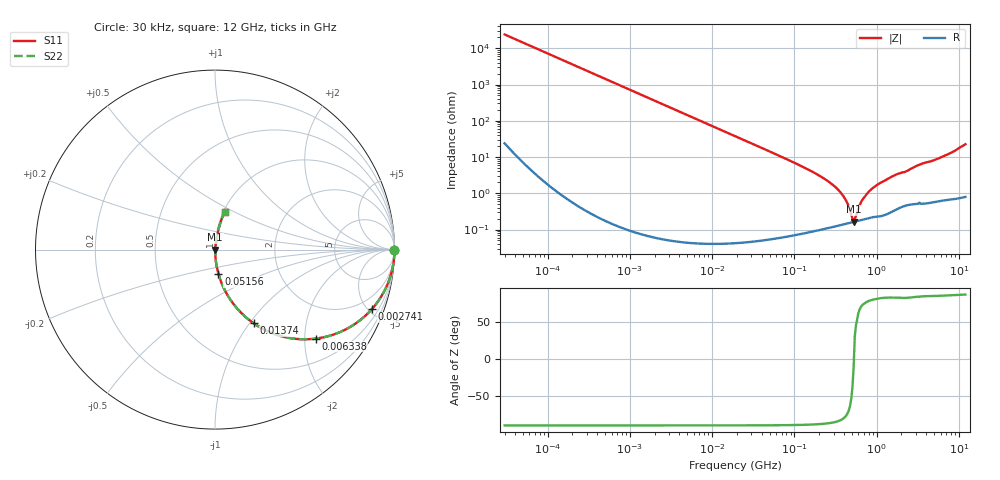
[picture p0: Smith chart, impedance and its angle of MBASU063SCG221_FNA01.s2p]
! MBASU063SCG221_FNA01  S-PARAMETER MODEL  ( General Type )
! Model Generated by TAIYO YUDEN Corporation (http://www.ty-top.com)
! Version 1.0
! TAIYO YUDEN Control No. 181120
! Copyright(c) 2018 TAIYO YUDEN CO.,LTD. All Rights Reserved.
! Product Description (link to TY-COMPAS)
! https://ds.yuden.co.jp/TYCOMPAS/or/detail?pn=MBASU063SCG221JFNA01&u=M
! Products Name : Multilayer Ceramic Capacitors
! Characteristics :
!  Capacitance : 220 pF , Rated Voltage : 50V , TCC : CG / C0G
!  Case Size : 0.6 x 0.3 / 0.024 x 0.012 [mm/inch] , Thickness : 0.3 / 0.012 [mm/inch]
!  (Conditions: Temperature = 25 degC , DC Bias Current/Voltage = 0A / 0V)
! External Node Assignments :
!  1  o---| |---o  2
! GND o---------o GND
! Frequency Range : 0.03MHz  -  12000MHz  [ 401 STEP ]
# MHz S RI R 50
! Freq[MHz].  S11 Real  S11 Imag  S21 Real  S21 Imag  S12 Real  S12 Imag  S22 Real  S22 Imag
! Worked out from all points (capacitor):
!   401 points, 30 kHz to 12 GHz, reference 50 ohm
!   read as one part in series: C = 221 pF near 32 kHz
!   lowest |Z| = 165 mohm at 525.6 MHz (marker M1)
!   series resonance near 529.5 MHz, so ESL is about 410 pH
!   S11 on the Smith chart (normalised r, x): 30 kHz: open; 2.741 MHz: 1.00, -5.25; 6.338 MHz: 1.00, -2.27; 13.74 MHz: 1.00, -1.05; 51.56 MHz: 1.00, -0.28; 12 GHz: 1.02, +0.45
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0.03  1 -0.00417  2.15e-05 0.00417  2.15e-05 0.00417  1 -0.00417
0.260295  0.9987 -0.0361  0.00131 0.0361  0.00131 0.0361  0.9987 -0.0361
0.858335  0.986 -0.1175  0.014 0.1175  0.014 0.1175  0.986 -0.1175
2.258455  0.9104 -0.2855  0.0896 0.2855  0.0896 0.2855  0.9104 -0.2855
2.740579  0.8734 -0.3324  0.1266 0.3324  0.1266 0.3324  0.8734 -0.3324
6.338349  0.5633 -0.4958  0.4367 0.4958  0.4367 0.4958  0.5633 -0.4958
13.74358  0.2153 -0.4107  0.7847 0.4107  0.7847 0.4107  0.2153 -0.4107
18.97367  0.1259 -0.3312  0.8741 0.3312  0.8741 0.3312  0.1259 -0.3312
51.55976  0.0193 -0.1356  0.9807 0.1356  0.9807 0.1356  0.0193 -0.1356
164.6252  0.00243 -0.0394  0.9976 0.0394  0.9976 0.0394  0.00243 -0.0394
258.5642  0.00155 -0.0212  0.9985 0.0212  0.9985 0.0212  0.00155 -0.0212
345.6326  0.00143 -0.012  0.9986 0.012  0.9986 0.012  0.00143 -0.012
419.4166  0.00147 -0.00648  0.9985 0.00648  0.9985 0.00648  0.00147 -0.00648
492.8008  0.00156 -0.00207  0.9984 0.00207  0.9984 0.00207  0.00156 -0.00207
525.6319  0.00162 -0.000291  0.9984 0.000291  0.9984 0.000291  0.00162 -0.000291
560.6502  0.00168 0.00173  0.9983 -0.00173  0.9983 -0.00173  0.00168 0.00173
658.7456  0.00187 0.00591  0.9981 -0.00591  0.9981 -0.00591  0.00187 0.00591
799.3715  0.00217 0.0108  0.9978 -0.0108  0.9978 -0.0108  0.00217 0.0108
1428.372  0.00353 0.0263  0.9965 -0.0263  0.9965 -0.0263  0.00353 0.0263
3303.507  0.00914 0.0602  0.9909 -0.0602  0.9909 -0.0602  0.00914 0.0602
5902.934  0.0149 0.0932  0.9851 -0.0932  0.9851 -0.0932  0.0149 0.0932
12000  0.0551 0.2111  0.9449 -0.2111  0.9449 -0.2111  0.0551 0.2111
